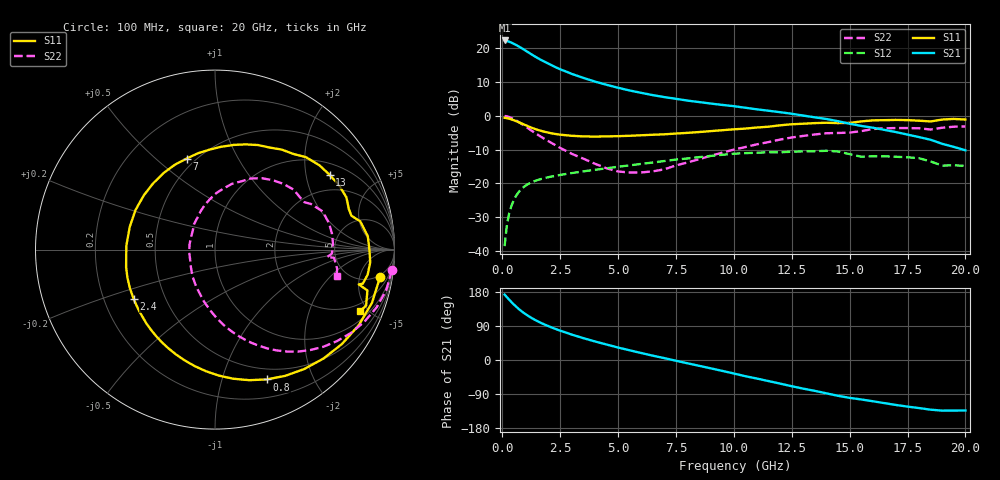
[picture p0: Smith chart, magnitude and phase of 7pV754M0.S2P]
! Infineon Technologies  Discrete & RF Semiconductors
! bfp620
! VCE = 0.75 V,  IC =  4.0 mA
! Common Emitter S-Parameters:  Sep 2002
# GHz  S  MA  R  50
!  f  S11  S21  S12  S22
! GHz  MAG  ANG  MAG  ANG  MAG  ANG  MAG  ANG
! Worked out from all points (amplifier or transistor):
!   59 points, 100 MHz to 20 GHz, reference 50 ohm
!   highest |S21| = 22.3 dB at 100 MHz (marker M1)
!   |S21| within 3 dB of that: start of sweep to 1.003 GHz
!   unconditionally stable (mu >= 1): 5.109 GHz to 11.8 GHz; 14.68 GHz to 15.56 GHz; 16.77 GHz to end of sweep
!   at 1 GHz: K = 0.28, MSG = 20.0 dB, |S12| = -20.7 dB
!   at 5.5 GHz: K = 1.03, MAG = 10.0 dB, |S12| = -14.7 dB
!   at 20 GHz: K = 1.62, MAG = -2.3 dB, |S12| = -14.9 dB
!   S11 on the Smith chart (normalised r, x): 100 MHz: 4, -10; 800 MHz: 0.38, -1.40; 2.4 GHz: 0.33, -0.25; 7 GHz: 0.45, +0.63; 13 GHz: 1.38, +2.74; 20 GHz: 1.47, -4.43
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0.1  0.9322 -9.5  13.05 172.5  0.0117 80.8  0.9922 -6.7
0.2  0.9235 -18.7  12.83 165.7  0.0244 79.8  0.9805 -13.3
0.3  0.9049 -27.7  12.49 159.0  0.0361 75.1  0.9563 -19.7
0.5  0.8566 -45.1  11.63 146.4  0.0567 65.5  0.8885 -31.5
0.7  0.8046 -61.0  10.69 135.2  0.0735 57.4  0.8108 -41.9
0.8  0.7783 -68.3  10.21 130.2  0.0805 53.8  0.7714 -46.5
0.9  0.7522 -75.3  9.725 125.5  0.0866 50.5  0.7324 -50.9
1.1  0.7025 -88.2  8.8 117.1  0.0967 44.9  0.6579 -58.6
1.3  0.6588 -99.9  7.966 109.7  0.1046 40.3  0.5905 -65.3
1.5  0.623 -110.5  7.249 103.1  0.111 36.5  0.5318 -71.3
1.9  0.5713 -128.8  6.128 91.7  0.121 30.8  0.4385 -81.6
2.4  0.5305 -148.7  5.058 79.6  0.131 25.5  0.3495 -93.0
3  0.505 -168.7  4.17 67.0  0.1415 20.5  0.273 -106.1
3.5  0.4945 177.6  3.643 57.7  0.1502 17.1  0.2315 -116.9
5  0.4986 142.7  2.599 32.9  0.1756 7.7  0.1495 -157.9
7  0.5313 107.3  1.89 4.9  0.2134 -5.5  0.161 140.7
8.5  0.5741 86.5  1.597 -15.3  0.244 -17.5  0.2271 110.9
10.5  0.6458 61.6  1.314 -42.8  0.2796 -37.4  0.3442 82.0
13  0.7627 33.1  1.006 -75.6  0.2967 -61.8  0.5032 50.2
13.5  0.7783 27.5  0.948 -81.5  0.2987 -67.0  0.5283 43.9
17  0.8676 -4.7  0.573 -118.7  0.247 -97.3  0.6577 7.7
20  0.8785 -23.1  0.308 -133.2  0.1805 -112.7  0.6937 -12.1
